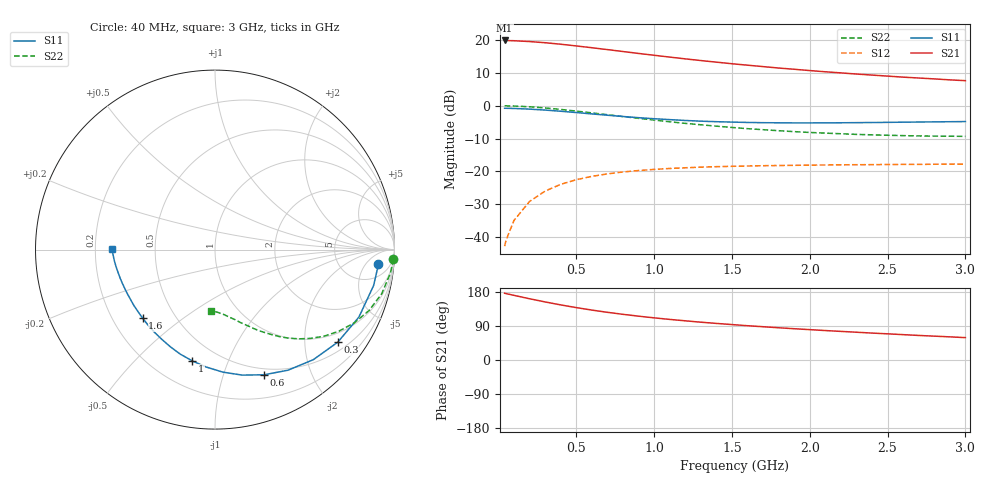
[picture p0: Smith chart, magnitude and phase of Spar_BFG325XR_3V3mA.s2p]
! Filename: 33BFG325XR.s2p
! Title: BFG325XR,RN20042071,Lot:TT3899C,B:Y13641,Sl.:1
! Bias: VCE=2.999V; IC=2.974mA;
! Company: NXP Semiconductors NL
! User: Q&R DSC-N
! Measure time: 29 Mar 2004 / 13:38:09
#  MHz  S  MA  R 50
! Freq  S11  S21  S12  S22  :
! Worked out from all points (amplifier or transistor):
!   32 points, 40 MHz to 3 GHz, reference 50 ohm
!   highest |S21| = 19.8 dB at 40 MHz (marker M1)
!   |S21| within 3 dB of that: start of sweep to 737.8 MHz
!   unconditionally stable (mu >= 1): nowhere
!   at 400 MHz: K = 0.17, MSG = 21.3 dB, |S12| = -23.9 dB
!   at 1.5 GHz: K = 0.57, MSG = 15.6 dB, |S12| = -18.4 dB
!   at 3 GHz: K = 0.92, MSG = 12.7 dB, |S12| = -17.8 dB
!   S11 on the Smith chart (normalised r, x): 40 MHz: 11, -11; 300 MHz: 0.73, -2.82; 600 MHz: 0.43, -1.37; 1 GHz: 0.36, -0.75; 1.6 GHz: 0.33, -0.36; 3 GHz: 0.27, +0.00
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40  0.9125 -5.1  9.787 176.1  0.00732 86.9  0.9945 -3.0
50  0.9119 -6.4  9.766 175.2  0.009091 86.1  0.9936 -3.8
100  0.9062 -12.7  9.69 170.6  0.01796 82.1  0.9863 -7.5
200  0.8856 -25.1  9.417 161.7  0.03494 74.9  0.961 -14.8
300  0.8567 -37.0  9.042 153.2  0.05028 68.2  0.9228 -21.6
400  0.8224 -48.2  8.582 145.4  0.0636 62.0  0.8763 -27.8
500  0.7854 -58.8  8.083 138.3  0.07488 56.6  0.8264 -33.4
600  0.7489 -68.7  7.59 131.8  0.08416 51.8  0.7765 -38.4
700  0.7154 -77.8  7.108 125.9  0.0918 47.6  0.728 -42.8
800  0.6842 -86.3  6.643 120.5  0.09818 44.0  0.6829 -46.7
900  0.6563 -94.2  6.216 115.7  0.1032 40.8  0.6413 -50.3
1000  0.6328 -101.6  5.829 111.2  0.1074 38.1  0.604 -53.4
1100  0.6134 -108.5  5.47 107.1  0.1109 35.7  0.569 -56.3
1200  0.5955 -114.8  5.141 103.4  0.1137 33.6  0.5382 -59.1
1300  0.5809 -120.8  4.847 99.8  0.1162 31.8  0.512 -61.7
1400  0.5706 -126.4  4.582 96.6  0.1182 30.3  0.488 -64.0
1600  0.5556 -136.5  4.122 90.5  0.121 27.7  0.4469 -68.6
1800  0.5488 -145.4  3.729 85.1  0.1231 25.9  0.4162 -72.6
2100  0.5475 -156.7  3.27 77.7  0.1254 23.8  0.3824 -78.5
2400  0.5538 -165.8  2.915 71.0  0.1268 22.7  0.36 -84.0
2600  0.5605 -171.1  2.712 66.9  0.1278 22.4  0.3502 -87.3
3000  0.5728 179.9  2.397 59.0  0.1295 21.8  0.3413 -94.1
